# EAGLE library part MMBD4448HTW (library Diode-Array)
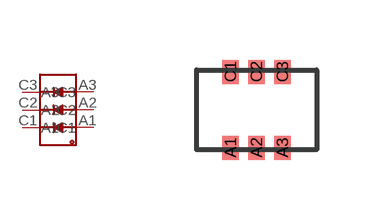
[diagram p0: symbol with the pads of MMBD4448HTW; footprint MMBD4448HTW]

Designator prefix -

## MMBD4448HTW  [MMBD4448HTW]
A1  A1
A2  A2
A3  A3
C1  C1
C2  C2
C3  C3

## Footprint MMBD4448HTW (pad centres in mm)
smd 0.42 x 0.6: A1 -0.65,-0.95; A2 0,-0.95; A3 0.65,-0.95; C1 -0.65,0.95; C2 0,0.95; C3 0.65,0.95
